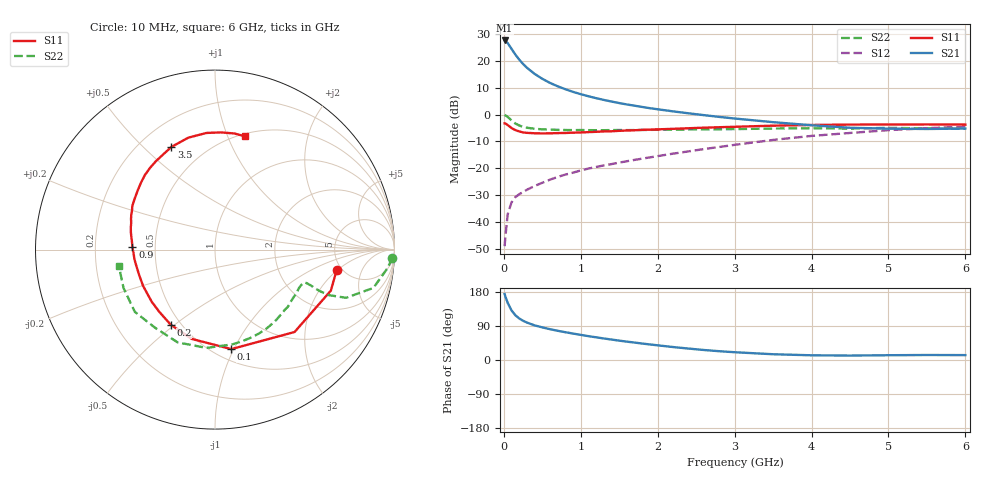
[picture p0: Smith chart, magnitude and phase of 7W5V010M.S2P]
! Infineon Technologies  Discrete & RF Semiconductors
! BFS17W
! Si NPN RF Bipolar Junction Transistor in SOT323
! VCE = 5 V  IC = 10 mA
! Common Emitter S-Parameters:  August  1999
# GHz  S  MA  R  50
!  f  S11  S21  S12  S22
! GHz  MAG  ANG  MAG  ANG  MAG  ANG  MAG  ANG
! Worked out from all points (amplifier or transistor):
!   36 points, 10 MHz to 6 GHz, reference 50 ohm
!   highest |S21| = 27.7 dB at 10 MHz (marker M1)
!   |S21| within 3 dB of that: start of sweep to 96.89 MHz
!   unconditionally stable (mu >= 1): 413.2 MHz to 2.328 GHz; 5.145 GHz to end of sweep
!   at 250 MHz: K = 0.79, MSG = 23.9 dB, |S12| = -28.9 dB
!   at 1.4 GHz: K = 1.19, MAG = 9.0 dB, |S12| = -18.5 dB
!   at 6 GHz: K = 1.05, MAG = -1.8 dB, |S12| = -4.5 dB
!   S11 on the Smith chart (normalised r, x): 10 MHz: 4.49, -1.97; 100 MHz: 0.60, -0.98; 200 MHz: 0.44, -0.48; 900 MHz: 0.37, +0.01; 3.5 GHz: 0.33, +0.61; 6 GHz: 0.53, +1.16
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0.01  0.687 -9.7  24.25 174.0  0.0035 81.0  0.9888 -2.6
0.02  0.6848 -19.5  23.97 167.5  0.0052 84.0  0.9681 -6.0
0.05  0.6382 -46.0  21.66 150.8  0.0138 71.7  0.908 -13.6
0.1  0.5618 -80.7  16.9 130.9  0.023 59.9  0.7781 -20.2
0.15  0.5142 -104.6  13.2 117.9  0.0288 54.8  0.6829 -21.8
0.2  0.4858 -120.5  10.65 109.6  0.0327 55.6  0.6271 -21.6
0.25  0.4653 -131.9  8.813 103.5  0.0358 53.7  0.5908 -21.0
0.3  0.4567 -140.7  7.497 98.8  0.0396 55.9  0.5701 -20.5
0.4  0.4489 -153.3  5.76 91.4  0.0465 58.3  0.5436 -20.1
0.5  0.4456 -161.6  4.665 86.0  0.0534 60.8  0.5318 -20.2
0.6  0.4474 -167.9  3.907 81.3  0.0611 62.6  0.5243 -21.0
0.7  0.452 -173.2  3.38 77.1  0.0686 64.0  0.5196 -22.3
0.9  0.4607 178.4  2.659 69.8  0.0826 66.0  0.5136 -25.4
1.1  0.4714 171.4  2.202 62.9  0.0984 66.8  0.5131 -29.3
1.3  0.4855 165.1  1.881 56.8  0.1128 67.7  0.5119 -33.8
1.6  0.5062 157.1  1.547 48.4  0.135 69.0  0.5136 -40.8
2.2  0.5427 142.4  1.15 34.2  0.1868 70.4  0.5249 -56.7
2.8  0.5819 128.4  0.907 23.2  0.2489 69.0  0.5328 -73.9
3.5  0.6217 113.0  0.723 15.2  0.337 64.2  0.5497 -94.9
4.5  0.6517 94.2  0.568 11.7  0.4544 52.0  0.5487 -127.5
5.5  0.656 80.5  0.539 13.2  0.5574 39.0  0.5528 -157.2
6  0.6526 75.2  0.55 12.9  0.5985 32.7  0.5434 -170.3
